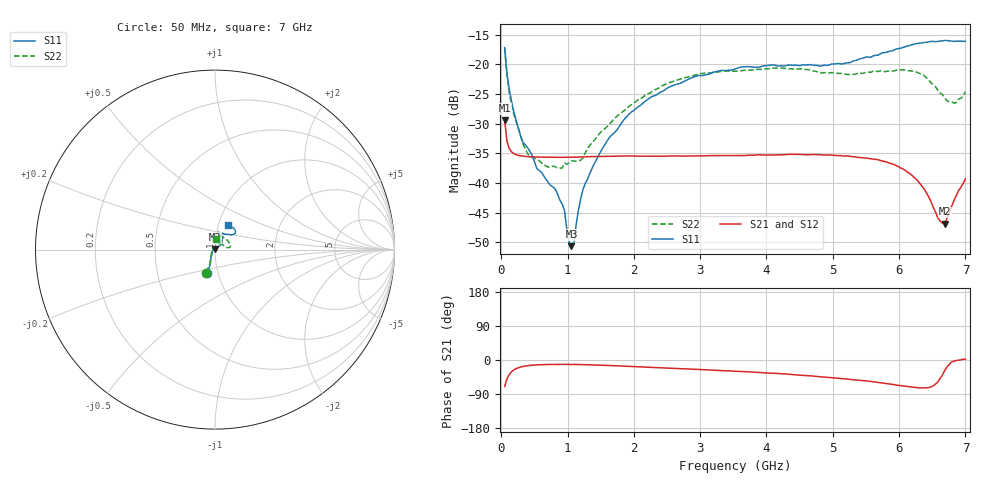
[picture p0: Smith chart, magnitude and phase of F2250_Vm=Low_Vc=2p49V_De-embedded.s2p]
! Integrated Device Technology
! Corporate Headquarters
! 6024 Silver Creek Valley Road
! San Jose, CA 95138  USA
! Phone:  1-408-284-8200
! Toll Free:  1-800-223-1366
! Webpage:  http://www.idt.com/
! Timing and RF Division
! 515 Groton Road, Suite 102
! Westford, MA 01886-6024
! Device:  F2250
! Description: Voltage Variable RF Attenuator
! Frequency:  50.0 -  6000.00 MHz
! Package:  3x3 mm Thin QFN Plastic Package: 16 pin
! Ports:  2 RF, 3 DC
!  Pin  1  = GND
!  Pin  2  = NC
!  Pin  3  = RF1  = Port 1
!  Pin  4  = NC
!  Pin  5  = GND
!  Pin  6  = GND
!  Pin  7  = GND
!  Pin  8  = GND
!  Pin  9  = NC
!  Pin 10  = RF2  = Port 2
!  Pin 11  = NC
!  Pin 12  = GND
!  Pin 13  = GND
!  Pin 14  = VCNTRL
!  Pin 15  = VDD
!  Pin 16  = VMODE
! Vcntrl:  2.490 Volts
! Vmode:  +0.000 Volts
! Vdd:  +3.30  Volts
! Current:  1.175 mA
! Data:  The device was measured on a the F2250 evaluation board which has
!  individual transmission lines to the RF pins.  Data was collected
!  using a calibrated network analyzer.  The evaluation board was
!  de-embedded using a TRL calibration technique.
!  The reference plane is the edge of the package pin.
! Misc:  SN 10
!  Action Tracker AT0258
! Date Measured:  2014-11-26
! Date:  2015-10-15  MJV
! Note:
!  Integrated Device Technology supplies this data as a sample of measured
!  data at the package pin for this product.  Your particular data for this
!  product may vary.
!  Data was taken at 25 degrees C.
!  Integrated Device Technology reserves the right to change this data at anytime.
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# GHz S dB R 50
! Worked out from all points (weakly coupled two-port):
!   201 points, 50 MHz to 7 GHz, reference 50 ohm
!   highest |S21| = -29.41 dB at 50 MHz (marker M1); lowest = -46.9 dB at 6.687 GHz (marker M2)
!   lowest |S11| = -50.7 dB at 1.058 GHz (marker M3), VSWR 1.01, Z = 49.8 + j0.246 ohm
!   |S11| at or under -10 dB: start of sweep to end of sweep
!   |S22| runs from -37.5 to -17.3 dB; largest |S21 - S12| = 6.7e-05
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0.05  -17.18 -108.6  -29.41 -69.8  -29.41 -69.8  -17.28 -111.0
0.08475  -21.45 -107.4  -32.92 -50.4  -32.92 -50.3  -21.75 -110.2
0.15425  -26.23 -116.6  -34.75 -31.1  -34.75 -31.2  -26.81 -122.4
0.29325  -32.20 -127.6  -35.43 -18.5  -35.43 -18.5  -32.10 -137.5
0.3975  -34.09 -141.8  -35.56 -15.0  -35.56 -15.0  -35.05 -160.4
0.5365  -37.57 -155.6  -35.64 -12.9  -35.63 -12.8  -36.04 178.2
0.91875  -43.54 158.1  -35.69 -11.5  -35.69 -11.5  -37.49 133.5
0.9535  -44.65 169.6  -35.68 -11.5  -35.68 -11.5  -36.66 131.3
1.023  -50.05 144.2  -35.67 -11.6  -35.67 -11.6  -36.62 115.9
1.05775  -50.65 122.7  -35.67 -11.6  -35.67 -11.6  -36.28 110.8
1.0925  -50.36 89.5  -35.65 -11.7  -35.66 -11.7  -36.30 106.3
1.162  -44.67 56.8  -35.64 -11.8  -35.64 -11.8  -36.25 95.6
1.2315  -41.11 44.2  -35.61 -12.1  -35.61 -12.1  -35.79 85.9
1.6485  -32.12 41.9  -35.52 -14.6  -35.52 -14.6  -29.87 64.6
2.37825  -24.87 47.3  -35.48 -20.3  -35.48 -20.3  -23.99 56.8
3.525  -20.80 72.4  -35.41 -29.5  -35.40 -29.5  -21.19 74.8
4.7065  -20.16 72.3  -35.21 -42.5  -35.20 -42.6  -21.15 72.3
5.85325  -17.81 40.5  -36.64 -63.3  -36.64 -63.3  -21.13 23.0
6.27025  -16.50 40.1  -39.49 -72.6  -39.50 -72.6  -21.35 9.6
6.68725  -15.99 48.8  -46.86 -27.7  -46.82 -27.4  -25.65 28.5
6.861  -16.13 55.1  -42.18 -1.3  -42.13 -1.2  -26.47 58.0
7  -16.12 63.2  -39.34 1.9  -39.29 1.7  -24.63 83.1
